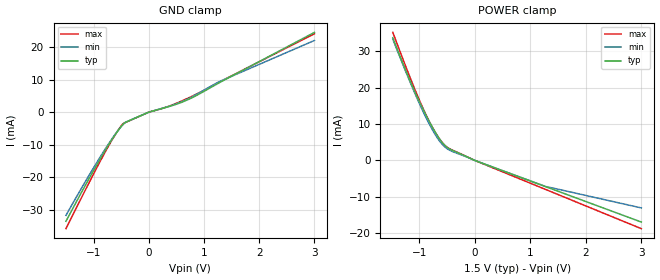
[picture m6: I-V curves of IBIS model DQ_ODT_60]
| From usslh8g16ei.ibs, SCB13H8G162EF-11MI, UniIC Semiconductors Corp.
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|   Model DQ_ODT_60
[Model] DQ_ODT_60
Model_type Input
Polarity   Non-Inverting
Enable   Active-High
Vinl =  0.615V
Vinh =  0.885V
C_comp   1.039pF   1.021pF   1.052pF
C_comp_power_clamp   0.685pF   0.671pF   0.699pF
C_comp_gnd_clamp   0.354pF   0.351pF   0.354pF
[Model Spec]
Vinh   0.885V   0.776V   0.922V
Vinl   0.615V   0.506V   0.652V
[Temperature Range]   45.000   95.000   -40.000
[Voltage Range]   1.500V   1.283V   1.575V
[C Comp Corner]
C_comp_power_clamp   0.699pF   0.671pF   0.685pF
C_comp_gnd_clamp   0.354pF   0.351pF   0.354pF
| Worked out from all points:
|   GND clamp passes 1 mA (typ) near -0.14 V on its own axis
|   POWER clamp passes 1 mA (typ) near -0.14 V on its own axis
[GND_clamp]
|Voltage   I(typ)   I(min)   I(max)
-1.5V     -33.55mA   -31.74mA   -35.82mA
-1.128V   -21.85mA   -20.74mA   -23.25mA
-818mV    -12.59mA   -12.1mA    -13.15mA
-632mV    -7.527mA   -7.358mA   -7.603mA
-477mV    -3.964mA   -3.994mA   -3.71mA
-415mV    -3.063mA   -3.05mA    -3.116mA
-12mV     -88.56uA   -88.18uA   -90.11uA
360mV     1.7mA      1.783mA    1.801mA
763mV     4.278mA    4.531mA    4.729mA
1.29V     9.168mA    9.48mA     9.365mA
3V        24.53mA    22.05mA    24.12mA
[POWER_clamp]
|Voltage   I(typ)   I(min)   I(max)
-1.476V   33.66mA    33.24mA    35.12mA
-1.166V   21.87mA    21.54mA    22.78mA
-1.011V   16.57mA    16.07mA    17.02mA
-887mV    12.67mA    12.02mA    12.78mA
-763mV    9.098mA    8.414mA    9.052mA
-670mV    6.717mA    6.088mA    6.68mA
-577mV    4.756mA    4.253mA    4.741mA
-484mV    3.44mA     3.072mA    3.469mA
12mV      -67.6uA    -67.19uA   -74.84uA
1.283V    -7.228mA   -7.184mA   -8.002mA
3V        -16.9mA    -13.03mA   -18.71mA
